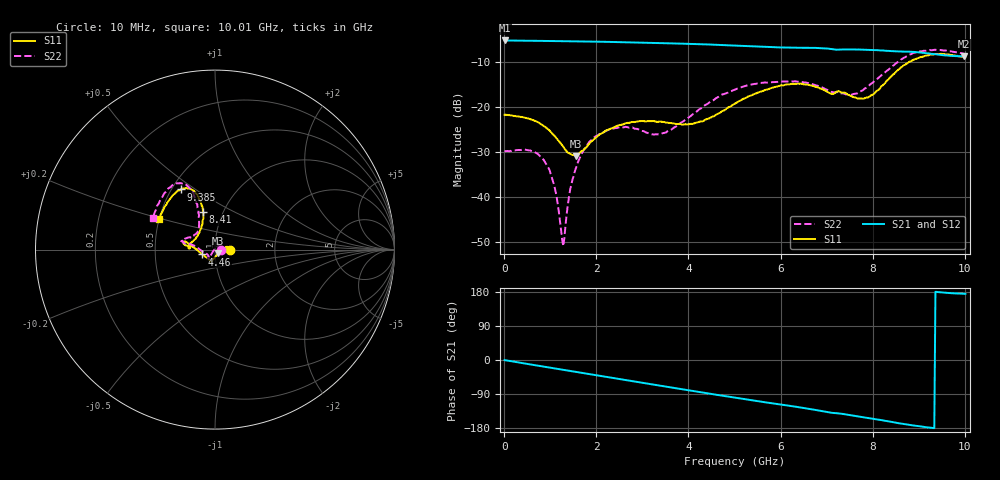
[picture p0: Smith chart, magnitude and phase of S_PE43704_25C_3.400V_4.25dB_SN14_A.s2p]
! Device ID: PE43704
! Dir: z:\PE43704\PE43704_Char_1_20130516\PE43704\AMB\3p400V\4p25dB
! Serial: 14
! Insertion: A
! Impedance: 50 ohm
! Temp: Amb
! VDD: 3.400V
! Attenuation Step: 4.25dB
! IDD: 1.140975e-01mA
#  Hz  S  RI  R  50
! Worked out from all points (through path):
!   401 points, 10 MHz to 10.01 GHz, reference 50 ohm
!   highest |S21| = -5.26 dB at 10 MHz (marker M1); lowest = -8.8 dB at 9.985 GHz (marker M2)
!   group delay of S21, straight-line fit = 52.9 ps
!   lowest |S11| = -30.9 dB at 1.56 GHz (marker M3), VSWR 1.06, Z = 51.9 - j2.25 ohm
!   |S11| at or under -10 dB: start of sweep to 8.791 GHz
!   |S22| runs from -50.9 to -7.3 dB; largest |S21 - S12| = 0.0037
!   S11 on the Smith chart (normalised r, x): 10 MHz: 1.18, +0.00; 4.46 GHz: 0.87, -0.05; 8.41 GHz: 0.80, +0.36; 9.385 GHz: 0.56, +0.44; 10.01 GHz: 0.50, +0.19
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1e7  0.0819 9.92e-05  0.5457 -0.00231  0.546 -0.00218  0.0322 0.000398
5.6e8  0.0718 0.0155  0.5306 -0.1079  0.5305 -0.1078  0.026 0.0202
8.6e8  0.0599 0.0137  0.5145 -0.1626  0.5145 -0.1625  0.0174 0.0191
1.085e9  0.0481 0.00578  0.4993 -0.2026  0.4992 -0.2023  0.0074 0.0115
1.235e9  0.0389 -0.00216  0.4865 -0.2284  0.4866 -0.2281  8.01e-05 0.00432
1.285e9  0.0358 -0.00511  0.4818 -0.2366  0.4818 -0.2365  -0.00255 0.00129
1.435e9  0.0262 -0.0148  0.4677 -0.261  0.4676 -0.2609  -0.00948 -0.00786
1.56e9  0.0186 -0.0216  0.455 -0.2807  0.4548 -0.2806  -0.0142 -0.0158
1.685e9  0.0118 -0.0303  0.441 -0.3  0.441 -0.2998  -0.0192 -0.0238
2.36e9  -0.013 -0.0572  0.3532 -0.3881  0.3534 -0.3881  -0.0336 -0.0464
3.36e9  -0.0264 -0.0633  0.1969 -0.4707  0.1975 -0.4704  -0.0399 -0.0295
4.46e9  -0.0704 -0.0267  0.00985 -0.4919  0.0102 -0.4922  -0.1112 0.0204
5.01e9  -0.1086 0.00479  -0.0773 -0.4722  -0.0769 -0.4726  -0.1531 0.0289
5.985e9  -0.1661 0.0449  -0.2084 -0.4071  -0.2064 -0.4076  -0.1847 0.0465
6.685e9  -0.1697 0.0279  -0.2924 -0.3441  -0.2926 -0.3436  -0.1687 0.0605
7.585e9  -0.1169 0.0521  -0.3643 -0.2365  -0.3637 -0.2359  -0.0961 0.1008
7.935e9  -0.0852 0.1  -0.3847 -0.1893  -0.3853 -0.1903  -0.089 0.1519
8.36e9  -0.0653 0.1964  -0.3975 -0.1268  -0.397 -0.1286  -0.098 0.2457
8.41e9  -0.0665 0.2106  -0.3985 -0.1193  -0.3981 -0.1206  -0.1039 0.2588
9.385e9  -0.1906 0.3355  -0.3823 0.00264  -0.3832 0.00405  -0.2434 0.3519
9.985e9  -0.3058 0.1806  -0.3611 0.0333  -0.3623 0.0341  -0.3406 0.1836
1.001e10  -0.3112 0.1697  -0.3622 0.0342  -0.3641 0.0341  -0.3438 0.1751
